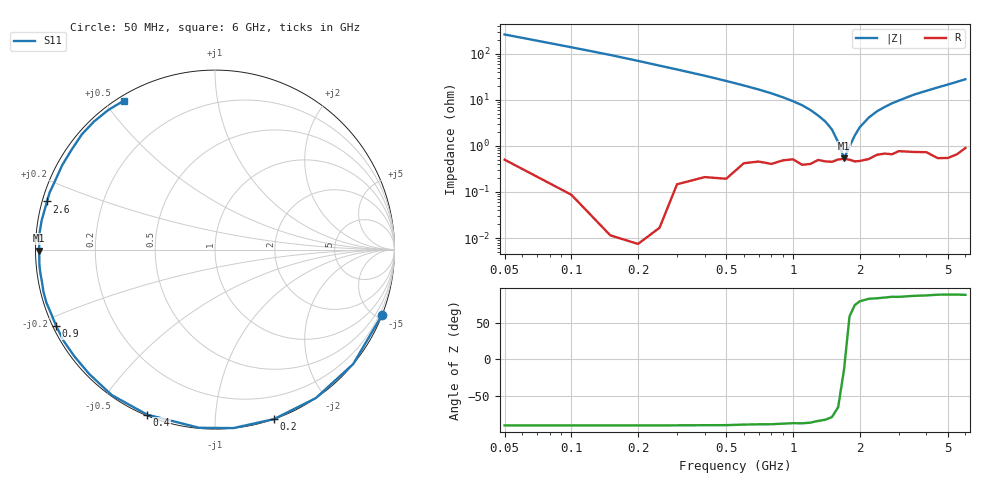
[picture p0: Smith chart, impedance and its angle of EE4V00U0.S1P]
! Infineon Technologies  Discrete & RF Semiconductors
! BBY55-02W
! Si Tuning Diode in SCD-80
! VR = 4 V
! S-Parameters:  June  2000
# GHz  S  MA  R  50
!  f  S11
! GHz  MAG  ANG
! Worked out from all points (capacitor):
!   34 points, 50 MHz to 6 GHz, reference 50 ohm
!   read as one part to ground: C = 11.4 pF near 50 MHz
!   lowest |Z| = 542 mohm at 1.7 GHz (marker M1)
!   series resonance near 1.714 GHz, so ESL is about 760 pH
!   S11 on the Smith chart (normalised r, x): 50 MHz: 0.01, -5.27; 200 MHz: 0.00, -1.41; 400 MHz: 0.00, -0.67; 900 MHz: 0.01, -0.23; 2.6 GHz: 0.01, +0.14; 6 GHz: 0.02, +0.56
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0.05  0.9993 -21.5
0.1  0.9996 -39.6
0.15  0.9999 -55.8
0.2  0.9999 -70.8
0.25  0.9997 -84.1
0.3  0.9968 -95.1
0.4  0.9942 -112.4
0.5  0.9939 -125.4
0.6  0.9857 -135.3
0.7  0.9837 -142.8
0.8  0.985 -149.0
0.9  0.9817 -154.3
1  0.9804 -158.8
1.1  0.9849 -162.6
1.2  0.9841 -166.3
1.3  0.9805 -169.6
1.6  0.9799 -177.5
1.7  0.9792 -179.7
2  0.9814 174.3
2.4  0.9748 167.1
2.6  0.9736 164.0
2.8  0.9747 160.9
3.5  0.9726 151.1
4  0.9737 145.1
4.5  0.9811 139.1
5  0.9817 133.4
5.5  0.979 127.4
6  0.9729 121.4
